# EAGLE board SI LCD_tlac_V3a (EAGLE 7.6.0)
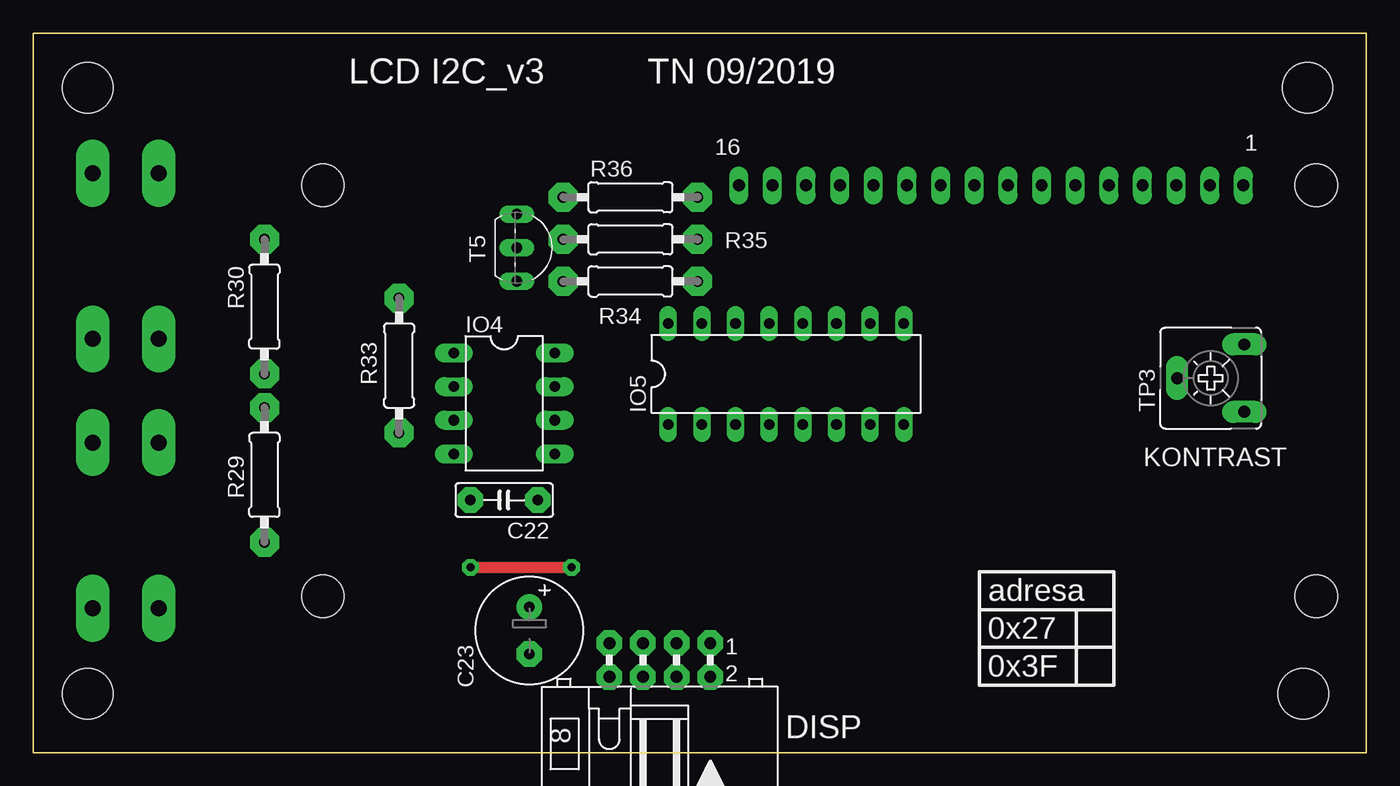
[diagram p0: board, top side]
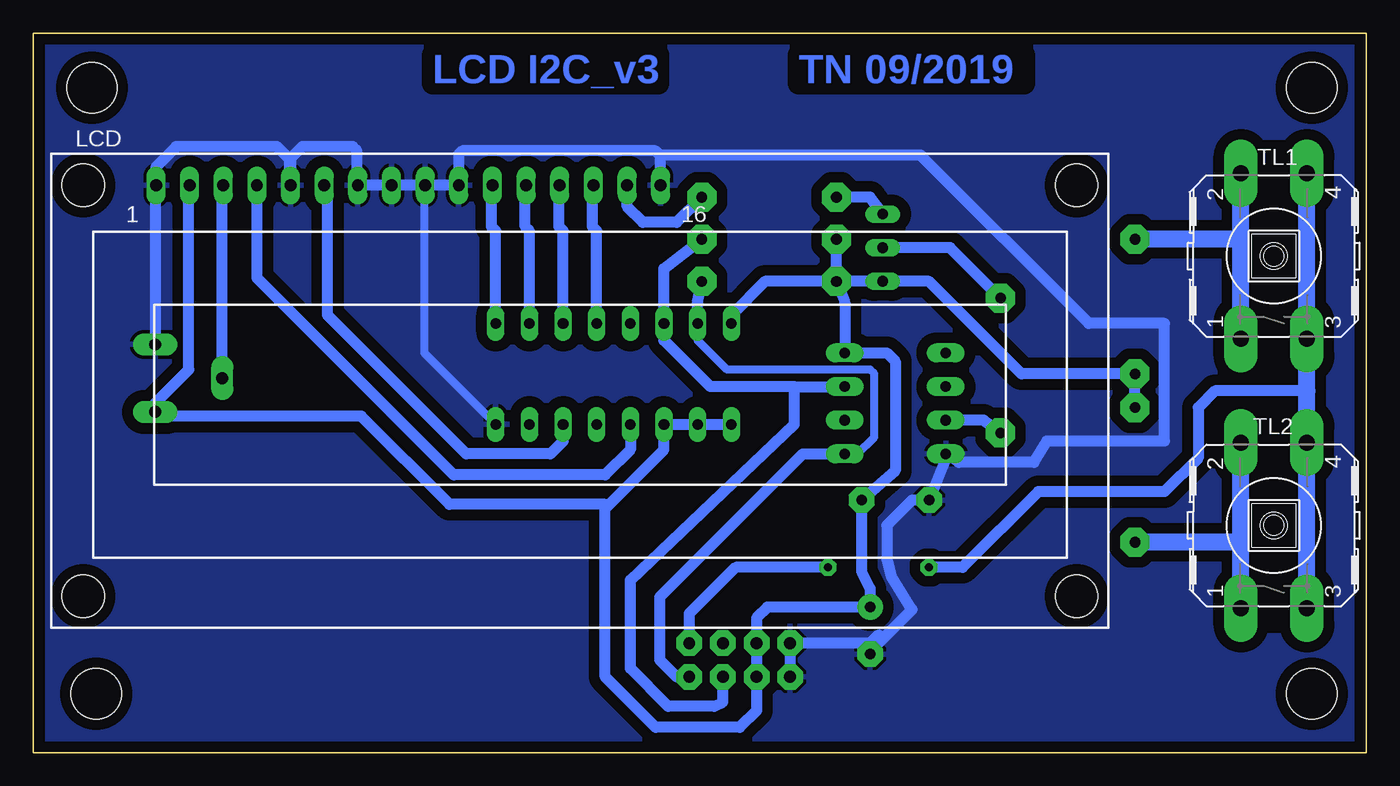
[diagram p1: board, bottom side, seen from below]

Size 100.65 x 54.29 mm. Coordinates in mm from the lower left corner, seen from the top.
Outline: 0,54.29 100.65,54.29 100.65,0 0,0 0,54.29
Copper layers (1*16): Top 0.035mm / dielectric 1.5mm / Bottom 0.035mm
Design rules "default *": minimum track width 10mil, minimum drill 24mil, track to track 8mil, track to pad 8mil, pad to pad 8mil, via to via 8mil, smd to smd 8mil, copper to edge 20mil, drill to drill 8mil, minimum pad ring 10mil, minimum via ring 8mil, stop-mask expansion 4mil, vias tented up to drill 0mil, thermal gap 10mil
Holes 3.8 mm at 4.13,4.45 4.13,50.16 96.2,50.16 95.89,4.45
bRestrict: area 5.7,9.8 to 8.3,45.4

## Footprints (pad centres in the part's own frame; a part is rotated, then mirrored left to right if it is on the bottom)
C050-025X075 = drill 0.8 pad 1.93 octagon: 1 -2.54,0; 2 2.54,0
E3,5-8 = drill 0.8 pad 1.93: + -1.778,0 | drill 0.8 pad 1.93 octagon: - 1.778,0
ML8L = drill 0.9 pad 1.93 octagon: 1 -5.08,-2.54; 2 -5.08,0; 3 -2.54,-2.54; 4 -2.54,0; 5 0,-2.54; 6 0,0; 7 2.54,-2.54; 8 2.54,0
DIL08 = drill 0.8 pad 1.422 long: 1 -3.81,-3.81; 2 -1.27,-3.81; 3 1.27,-3.81; 4 3.81,-3.81; 5 3.81,3.81; 6 1.27,3.81; 7 -1.27,3.81; 8 -3.81,3.81
DIL16 = drill 0.813 long: 1 -8.89,-3.81; 2 -6.35,-3.81; 3 -3.81,-3.81; 4 -1.27,-3.81; 5 1.27,-3.81; 6 3.81,-3.81; 7 6.35,-3.81; 8 8.89,-3.81; 9 8.89,3.81; 10 6.35,3.81; 11 3.81,3.81; 12 1.27,3.81; 13 -1.27,3.81; 14 -3.81,3.81; 15 -6.35,3.81; 16 -8.89,3.81
TUXGR_16X2_R2 = drill 0.9 pad 1.422 long: 1 -32,15.5; 2 -29.46,15.5; 3 -26.92,15.5; 4 -24.38,15.5; 5 -21.84,15.5; 6 -19.3,15.5; 7 -16.76,15.5; 8 -14.22,15.5; 9 -11.68,15.5; 10 -9.14,15.5; 11 -6.6,15.5; 12 -4.06,15.5; 13 -1.52,15.5; 14 1.02,15.5; 15 3.56,15.5; 16 6.1,15.5 | hole 3.2: -37.5,-15.5; 37.5,-15.5; -37.5,15.5; 37.5,15.5
0207/10 = drill 0.8 pad 2.184 octagon: 1 -5.08,0; 2 5.08,0
TO92-CBE = drill 0.813 long: B 0,0; C -2.54,0; E 2.54,0
RACON12 = drill 1.2 pad 2.54 long: 1 -6.248,2.489; 2 6.248,2.489; 3 -6.248,-2.489; 4 6.248,-2.489
CA6V = drill 0.9 pad 1.676 long: A -2.54,-2.54; E 2.54,-2.54; S 0,2.54

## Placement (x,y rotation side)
C22  100n  [C050-025X075]  35.56,19.05 180 top
C23  47u  [E3,5-8]  37.47,9.21 270 top
DISP  [ML8L]  46.04,5.71 180 top
IO4  Attiny85  [DIL08]  35.56,26.35 270 top
IO5  PCF8574P  [DIL16]  56.83,28.57 0 top
LCD  [TUXGR_16X2_R2]  59.37,27.3 0 bottom
R29  10k  [0207/10]  17.46,20.95 90 top
R30  5k6  [0207/10]  17.46,33.66 90 top
R33  1k  [0207/10]  27.62,29.21 270 top
R34  4k7  [0207/10]  45.09,35.56 0 top
R35  4k7  [0207/10]  45.09,38.73 0 top
R36  100  [0207/10]  45.09,41.91 0 top
T5  BC327  [TO92-CBE]  36.51,38.1 270 top
TL1  [RACON12]  6.99,37.47 90 bottom
TL2  [RACON12]  6.99,17.14 90 bottom
TP3  10k  [CA6V]  88.9,28.26 90 top

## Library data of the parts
C22 C23 = 12moje
DISP IO4 LCD R29 R30 R33-R36 TL1 TL2 TP3 = 11moje
IO5 = 40xx
T5 = transistor-neu-to92

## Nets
GND: C22.2 C23.- DISP.7 DISP.8 IO4.4 IO5.8 LCD.1 LCD.5 LCD.7 LCD.8 LCD.9 LCD.10 LCD.16 TP3.E
S$1: LCD.3 TP3.S
S$2: R36.1 T5.C
S$6: IO5.4 LCD.4
S$7: DISP.4 IO4.7 IO5.14 R35.2
S$10: IO5.6 LCD.6
S$11: IO5.9 LCD.11
S$12: IO5.10 LCD.12
S$13: IO5.11 LCD.13
S$14: IO5.12 LCD.14
S$15: LCD.15 R36.2
S$16: IO4.3 R33.2
S$20: DISP.2 IO4.5 IO5.15 R34.2
S$21: R30.2 TL1.1 TL1.2
S$22: DISP.1 TL1.3 TL1.4 TL2.3 TL2.4
S$25: R29.1 TL2.1 TL2.2
S$28: R33.1 T5.B
S$29: IO4.6
VCC: C22.1 C23.+ DISP.5 DISP.6 IO4.8 IO5.1 IO5.2 IO5.3 IO5.16 LCD.2 R29.2 R30.1 R34.1 R35.1 T5.E TP3.A

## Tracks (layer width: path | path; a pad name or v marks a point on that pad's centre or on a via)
GND
  Bottom 0.61: IO5.8 71.12,30.16 71.12,42.55 71.05,42.61 LCD.9 | LCD.16 53.27,44.84
  Bottom 0.813: TP3.E 91.44,42.86 91.38,42.8 LCD.1 91.37,44.2 89.85,45.72 82.23,45.72 81.28,44.77 81.28,42.86 81.22,42.8 LCD.5 81.21,44.84 80.33,45.72 76.52,45.72 76.2,45.4 76.2,42.86 76.14,42.8 LCD.7 73.72,42.8 73.66,42.86 73.6,42.8 LCD.8 71.18,42.8 71.12,42.86 71.06,42.8 LCD.9 LCD.10 | 68.26,42.86 68.32,42.8 LCD.10 | LCD.10 68.51,45.15 68.26,45.4 53.66,45.4 53.34,45.09 | 53.34,45.09 53.34,42.86 53.28,42.8 LCD.16 53.27,42.61 53.34,42.55 53.34,45.09 | DISP.8 DISP.7 37.47,8.26 36.83,8.89 C23.- 37.02,8.06 34.29,10.79 35.88,13.34 36.2,14.61 36.2,17.14 34.29,19.05 C22.2 31.75,22.23 IO4.4 30.8,21.91 25.08,21.91 24.13,23.5 15.24,23.5 15.24,32.38 20.95,32.38 33.66,45.09 53.34,45.09
  pour Bottom (isolate 0.813): 0,0 0,54.29 100.65,54.29 100.65,0
S$1
  Bottom 0.813: LCD.3 86.3,42.8 86.36,42.86 TP3.S
S$2
  Bottom 0.813: R36.1 37.47,41.91 T5.C
S$6
  Bottom 0.813: LCD.4 83.75,35.81 68.9,20.95 57.47,20.95 55.56,22.86 IO5.4
S$7
  Bottom 0.813: 43.18,27.62 IO4.7 | 43.18,27.62 49.53,27.62 53.02,31.11 IO5.14 53.02,36.51 R35.2 | DISP.4 48.58,3.81 49.21,3.49 52.7,3.49 55.56,6.35 55.56,13.02 43.18,24.77 43.18,27.62
S$10
  Bottom 0.813: 78.68,42.8 78.74,42.86 | 78.68,42.8 LCD.6 | 78.68,42.8 78.42,42.55 78.42,33.02 67.94,22.54 61.59,22.54 60.64,23.5 IO5.6
S$11
  Bottom 0.813: IO5.9 65.72,39.37 66.04,39.69 66.04,42.86 65.98,42.8 LCD.11
S$12
  Bottom 0.813: IO5.10 63.18,39.37 63.5,39.69 63.5,42.86 63.44,42.8 LCD.12
S$13
  Bottom 0.813: IO5.11 60.64,39.37 60.96,39.69 60.96,42.86 60.9,42.8 LCD.13
S$14
  Bottom 0.813: IO5.12 58.1,39.37 58.42,39.69 58.42,42.86 58.36,42.8 LCD.14
S$15
  Bottom 0.813: LCD.15 55.81,41.21 54.61,40.01 52.07,40.01 R36.2
S$16
  Bottom 0.813: IO4.3 28.89,25.08 R33.2
S$20
  Bottom 0.61: 50.48,31.43 50.48,31.11 48.26,28.89 37.47,28.89 37.15,28.57 37.15,23.81 38.42,22.54 39.05,22.54 39.37,22.23 IO4.5
  Bottom 0.813: 50.48,31.43 IO5.15 50.48,33.97 R34.2 | DISP.2 52.07,5.71 53.34,6.99 53.34,11.75 42.55,22.54 IO4.5
S$21
  Bottom 1.27: TL1.1 9.47,31.17 | 9.47,31.17 9.47,38.73 | 9.47,38.73 TL1.2 | 9.47,31.17 9.53,31.11 | 9.47,38.73 R30.2
S$22  (via drill 0.6 pad 1.27)
  Top 0.813: v33.02,13.97 v40.64,13.97
  Bottom 0.813: DISP.1 51.12,10.48 47.62,13.97 v40.64,13.97 | v33.02,13.97 30.48,13.97 24.77,19.68 15.24,19.68 12.7,22.23 12.7,26.04 11.43,27.3 4.5,27.3 4.45,27.3
  Bottom 1.27: TL1.3 4.5,31.17 4.45,31.11 | TL1.3 TL1.4 | TL2.4 4.5,27.3 TL1.3 | TL2.4 4.5,22.91 4.45,22.86 4.45,23.5 4.5,23.44 TL2.4 | TL2.3 4.5,10.85 | 4.5,10.85 TL2.4 | 4.5,10.85 4.45,10.79
S$25
  Bottom 1.27: TL2.1 9.47,10.85 | 9.47,10.85 9.47,15.88 | 9.47,15.88 TL2.2 | 9.47,10.85 9.53,10.79 | 9.47,15.88 R29.1
S$28
  Bottom 0.813: T5.B 31.43,38.1 R33.1
VCC
  Bottom 0.61: IO5.1 52.7,24.77
  Bottom 0.813: LCD.2 88.84,42.8 88.9,42.86 88.9,28.89 91.44,26.35 TP3.A 90.17,25.4 75.88,25.4 69.22,18.73 57.47,18.73 57.47,18.41 | IO5.16 47.94,33.02 45.4,35.56 R34.1 | R34.1 R35.1 | IO5.1 IO5.2 IO5.3 53.02,22.86 57.47,18.41 | 57.47,18.41 57.47,5.71 53.66,1.91 47.31,1.91 46.04,3.17 DISP.6 DISP.5 46.04,10.16 45.21,10.99 C23.+ 37.47,12.38 38.1,13.65 C22.1 35.56,21.27 35.56,29.53 36.2,30.16 IO4.8 39.37,33.97 R34.1 | R34.1 T5.E 33.02,35.56 26.04,28.57 R30.1 R29.2 17.14,26.04

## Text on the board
Bottom: TN 09/2019 | LCD I2C_v3
tNames: LCD I2C_v3 | TN 09/2019 | 16 | 1 | KONTRAST | adresa | 0x27 | 0x3F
